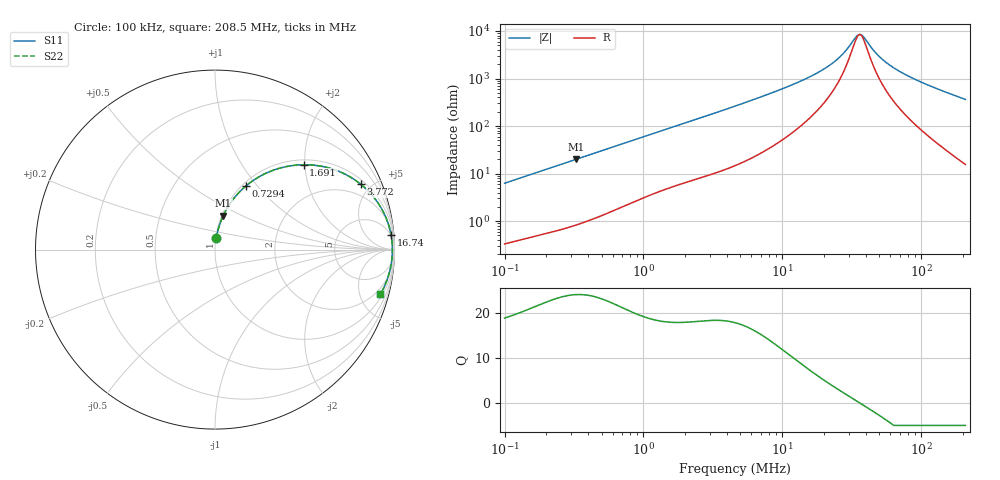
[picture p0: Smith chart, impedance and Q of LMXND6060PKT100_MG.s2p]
! LMXND6060PKT100_MG  S-PARAMETER MODEL  ( General Type )
! Model Generated by TAIYO YUDEN Corporation (https://www.yuden.co.jp/en/)
! Version 1.0
! TAIYO YUDEN Control No. 191025NI43SB-FBB
! Copyright(c) 2019 TAIYO YUDEN CO.,LTD. All Rights Reserved.
! Product Description (link to TY-COMPAS)
! https://ds.yuden.co.jp/TYCOMPAS/or/detail?pn=LMXND6060PKT100MMG&u=M
! Products Name : Inductors
! Characteristics :
!  Inductance : 10 uH , SRF(min) : 24 MHz , DC Resistance(max) : 0.168 Ohm
!  Rated Current : Saturation :1400 mA , Temp Rise : 1400 mA (40 degC)
!  Case Size : 6.0 x 6.0 / 0.236 x 0.236 [mm/inch] , Thickness : 1.4 / 0.055 [mm/inch]
!  (Conditions: Temperature = 25 degC , DC Bias Current/Voltage = 0A / 0V)
! External Node Assignments :
!  1  o---GGG---o  2
! GND o---------o GND
! Frequency Range : 0.1MHz  -  208.503118MHz  [ 402 STEP ]
# MHz S RI R 50
! Freq[MHz].  S11 Real  S11 Imag  S21 Real  S21 Imag  S12 Real  S12 Imag  S22 Real  S22 Imag
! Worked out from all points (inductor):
!   401 points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, 100 kHz to 208.5 MHz, reference 50 ohm
!   read as one part in series: L = 9.9 uH near 103.9 kHz
!   highest Q = 24.1 at 326.9 kHz (marker M1), where L = 9.72 uH
!   self-resonance near 35.95 MHz
!   S11 on the Smith chart (normalised r, x): 100 kHz: 1.01, +0.13; 729.4 kHz: 1.04, +0.88; 1.691 MHz: 1.11, +1.97; 3.772 MHz: 1.24, +4.33; 16.74 MHz: 5, +23; 208.5 MHz: 1.31, -7.27
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0.1  0.00718 0.062  0.9928 -0.062  0.9928 -0.062  0.00718 0.062
0.326936  0.0456 0.1889  0.9544 -0.1889  0.9544 -0.1889  0.0456 0.1889
0.359709  0.0537 0.2056  0.9463 -0.2056  0.9463 -0.2056  0.0537 0.2056
0.729406  0.1728 0.355  0.8272 -0.355  0.8272 -0.355  0.1728 0.355
1.293906  0.3747 0.4574  0.6253 -0.4574  0.6253 -0.4574  0.3747 0.4574
1.69072  0.4939 0.4728  0.5061 -0.4728  0.5061 -0.4728  0.4939 0.4728
2.43069  0.6553 0.4485  0.3447 -0.4485  0.3447 -0.4485  0.6553 0.4485
3.772059  0.8117 0.3646  0.1883 -0.3646  0.1883 -0.3646  0.8117 0.3646
4.654297  0.8645 0.3153  0.1355 -0.3153  0.1355 -0.3153  0.8645 0.3153
9.619882  0.9589 0.1619  0.0411 -0.1619  0.0411 -0.1619  0.9589 0.1619
16.42508  0.9807 0.0831  0.0193 -0.0831  0.0193 -0.0831  0.9807 0.0831
16.74193  0.9811 0.0807  0.0189 -0.0807  0.0189 -0.0807  0.9811 0.0807
21.05614  0.985 0.0542  0.015 -0.0542  0.015 -0.0542  0.985 0.0542
25.00684  0.9868 0.0361  0.0132 -0.0361  0.0132 -0.0361  0.9868 0.0361
28.58534  0.9877 0.0228  0.0123 -0.0228  0.0123 -0.0228  0.9877 0.0228
33.94871  0.9883 0.00608  0.0117 -0.00608  0.0117 -0.00608  0.9883 0.00608
35.95147  0.9883 0.00058  0.0117 -0.00058  0.0117 -0.00058  0.9883 0.00058
38.07238  0.9883 -0.00492  0.0117 0.00492  0.0117 0.00492  0.9883 -0.00492
47.88322  0.9877 -0.0272  0.0123 0.0272  0.0123 0.0272  0.9877 -0.0272
59.08252  0.986 -0.0489  0.014 0.0489  0.014 0.0489  0.986 -0.0489
97.09599  0.9762 -0.1095  0.0238 0.1095  0.0238 0.1095  0.9762 -0.1095
208.5031  0.9207 -0.2497  0.0793 0.2497  0.0793 0.2497  0.9207 -0.2497
